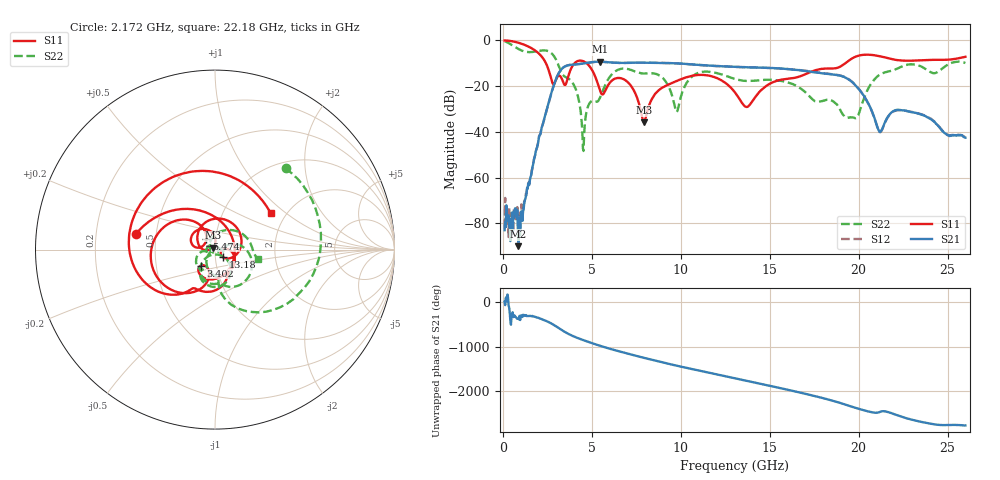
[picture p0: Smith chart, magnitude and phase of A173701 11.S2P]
!  2-Port S-parameters saved by WinCal
! VAR MeasName=S-Parameters (CALIBRATED_DATA) read from VNA (N5245A)
! VAR MeasDate=2017-6-7 10:29:08
! VAR NAME=A173701 11
! VAR FILENAME=A173701 11.S2P
! VAR DATE=2017-6-7 10:29:08
! VAR PHYS_PORTS=1,2
# Hz S DB R 50
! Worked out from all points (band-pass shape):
!   801 points, 100 MHz to 26 GHz, reference 50 ohm
!   highest |S21| = -9.30 dB at 5.442 GHz (marker M1); lowest = -90.0 dB at 877 MHz (marker M2)
!   |S21| within 3 dB of the highest: 3.334 GHz to 15.65 GHz (12.32 GHz wide, 130 % of centre)
!   lowest |S11| = -35.7 dB at 7.935 GHz (marker M3), VSWR 1.03, Z = 48.8 + j1.07 ohm
!   |S11| at or under -10 dB: 2.423 GHz to 4.028 GHz (1.605 GHz wide, 49.8 % of centre); 4.713 GHz to 19.25 GHz (14.53 GHz wide, 121 % of centre)
!   |S22| runs from -48.4 to -0.3 dB; largest |S21 - S12| = 0.0043
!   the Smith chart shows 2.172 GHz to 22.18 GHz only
!   S11 on the Smith chart (normalised r, x): 2.172 GHz: 0.38, +0.08; 3.402 GHz: 0.84, -0.15; 5.474 GHz: 0.90, +0.11; 13.18 GHz: 1.09, -0.09; 22.18 GHz: 1.66, +0.79
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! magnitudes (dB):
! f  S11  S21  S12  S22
! 100 MHz  0.0  -83.0  -82.1  -0.3
! 877 MHz  -1.0  -90.0  -77.0  -3.8
! 2.172 GHz  -6.9  -38.6  -38.6  -4.4
! 3.402 GHz  -18.4  -11.8  -11.8  -15.3
! 4.082 GHz  -9.6  -10.5  -10.5  -21.0
! 4.438 GHz  -8.9  -10.2  -10.2  -36.3
! 5.442 GHz  -21.4  -9.3  -9.3  -25.4
! 5.474 GHz  -22.2  -9.3  -9.3  -24.9
! 6.866 GHz  -17.3  -9.8  -9.9  -12.3
! 7.935 GHz  -35.7  -9.7  -9.7  -14.5
! 8.744 GHz  -21.9  -9.8  -9.8  -15.1
! 9.78 GHz  -17.7  -10.0  -10.1  -31.3
! 10.88 GHz  -15.2  -10.6  -10.7  -14.5
! 13.05 GHz  -22.7  -11.6  -11.6  -16.9
! 13.18 GHz  -24.2  -11.6  -11.6  -17.2
! 13.73 GHz  -29.1  -11.7  -11.7  -17.8
! 17.39 GHz  -13.5  -13.8  -13.7  -25.6
! 19.82 GHz  -7.1  -19.6  -19.5  -34.1
! 21.18 GHz  -6.9  -39.9  -40.1  -15.0
! 21.69 GHz  -7.9  -32.7  -33.0  -13.6
! 22.18 GHz  -8.6  -30.3  -30.6  -12.3
! 26 GHz  -7.2  -42.6  -42.7  -9.9
